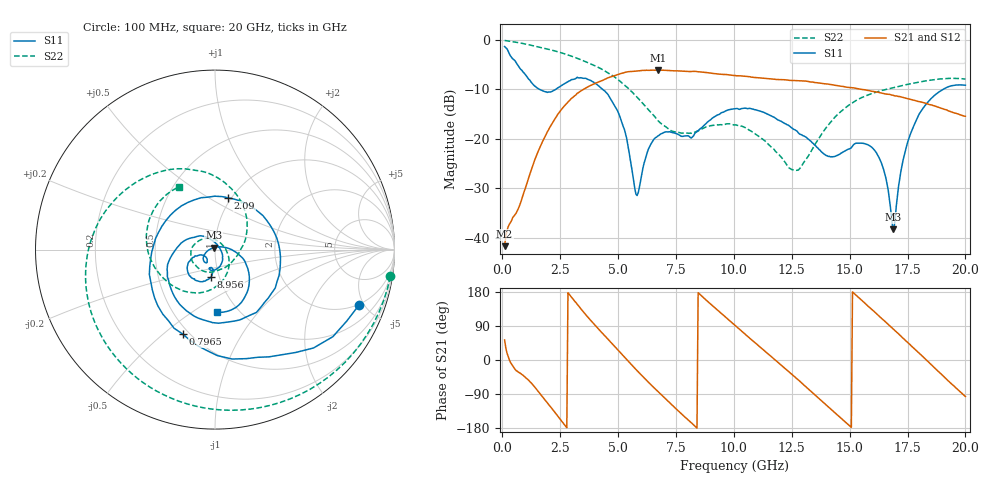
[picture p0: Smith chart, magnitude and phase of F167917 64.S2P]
!  2-Port S-parameters saved by WinCal
! VAR MeasName=S-Parameters (CALIBRATED_DATA) read from VNA (N5242A)
! VAR MeasDate=2016-11-22 9:03:13
! VAR NAME=F167917 64
! VAR FILENAME=F167917 64.S2P
! VAR DATE=2016-11-22 9:03:13
! VAR PHYS_PORTS=1,2
# Hz S DB R 50
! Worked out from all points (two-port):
!   401 points, 100 MHz to 20 GHz, reference 50 ohm
!   highest |S21| = -6.09 dB at 6.717 GHz (marker M1); lowest = -41.7 dB at 100 MHz (marker M2)
!   |S21| within 3 dB of the highest: 3.865 GHz to 14.3 GHz (10.43 GHz wide, 115 % of centre)
!   lowest |S11| = -38.3 dB at 16.87 GHz (marker M3), VSWR 1.02, Z = 49.3 + j1 ohm
!   |S11| at or under -10 dB: 1.611 GHz to 2.301 GHz (690.6 MHz wide, 35.3 % of centre); 4.338 GHz to 19.04 GHz (14.7 GHz wide, 126 % of centre)
!   |S22| runs from -26.4 to -0.1 dB; largest |S21 - S12| = 0.0049
!   S11 on the Smith chart (normalised r, x): 100 MHz: 1.92, -4.56; 796.5 MHz: 0.46, -0.58; 2.09 GHz: 0.97, +0.61; 8.956 GHz: 0.91, -0.28; 20 GHz: 0.80, -0.63
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1e8  -1.32 -21.2  -41.71 53.0  -41.75 54.6  -0.10 -8.7
7.965e8  -5.95 -110.8  -32.83 -35.6  -32.85 -35.1  -0.62 -63.3
1.3935e9  -9.30 176.1  -24.36 -70.7  -24.34 -70.4  -1.23 -103.4
2.09e9  -10.51 75.8  -17.37 -124.2  -17.37 -124.1  -2.00 -143.0
2.73675e9  -8.70 -6.4  -13.07 -174.9  -13.06 -174.6  -2.87 -175.0
3.43325e9  -7.69 -75.0  -10.19 132.1  -10.14 132.4  -4.08 154.2
4.9755e9  -14.31 169.3  -7.01 27.5  -6.98 27.2  -7.93 88.1
5.82125e9  -31.47 29.8  -6.28 -28.1  -6.28 -28.2  -11.57 49.7
6.71675e9  -19.41 -83.4  -6.09 -83.1  -6.09 -83.0  -16.28 6.5
6.7665e9  -19.31 -85.6  -6.09 -85.9  -6.10 -85.9  -16.51 4.2
7.91075e9  -19.40 -104.7  -6.34 -151.8  -6.32 -151.8  -18.80 -60.5
8.9555e9  -16.27 -98.6  -6.67 149.8  -6.64 149.8  -17.38 -115.7
1.005e10  -13.92 -121.2  -7.18 91.4  -7.16 91.5  -17.18 -164.3
1.169175e10  -15.52 -153.1  -7.91 5.1  -7.86 4.9  -21.96 128.7
1.268675e10  -18.32 -160.8  -8.22 -47.3  -8.21 -47.7  -26.37 45.4
1.338325e10  -20.78 -160.8  -8.50 -85.8  -8.49 -85.8  -22.14 -21.9
1.467675e10  -22.77 -126.8  -9.37 -156.2  -9.38 -156.3  -14.28 -83.3
1.59205e10  -21.58 -142.0  -10.34 135.3  -10.35 135.5  -10.88 -125.1
1.67165e10  -32.12 171.4  -11.00 91.3  -11.08 91.6  -9.85 -147.0
1.686575e10  -38.31 123.4  -11.17 82.7  -11.17 83.3  -9.68 -150.8
1.801e10  -14.93 -21.6  -12.48 17.9  -12.40 18.2  -8.50 179.8
2e10  -9.14 -88.3  -15.42 -96.3  -15.25 -96.4  -7.92 120.0
